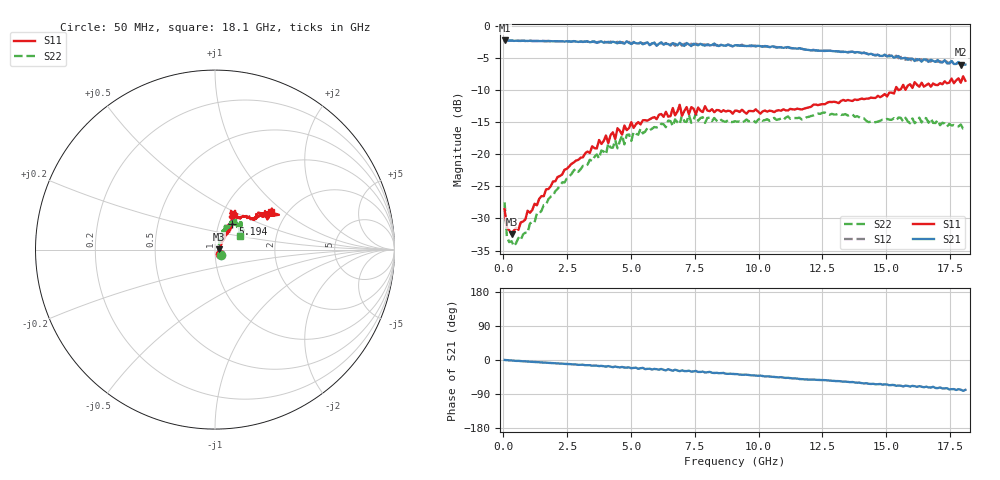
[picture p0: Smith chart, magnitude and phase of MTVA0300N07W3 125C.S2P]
! Network Analyzer HP8720D.06.14 Serial No. US36140669
!  7 Jul 2005  12:08:13
! Frequency  S11  S21  S12  S22
# HZ  S  DB R 50
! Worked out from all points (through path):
!   201 points, 50 MHz to 18.1 GHz, reference 50 ohm
!   highest |S21| = -2.25 dB at 50 MHz (marker M1); lowest = -6.0 dB at 17.92 GHz (marker M2)
!   group delay of S21, straight-line fit = 12.2 ps
!   lowest |S11| = -32.5 dB at 320.8 MHz (marker M3), VSWR 1.05, Z = 52.4 + j0.113 ohm
!   |S11| at or under -10 dB: start of sweep to 15.35 GHz
!   |S22| runs from -34.3 to -13.5 dB; largest |S21 - S12| = 0.042
!   S11 on the Smith chart (normalised r, x): 50 MHz: 1.06, -0.05; 5.194 GHz: 1.16, +0.34; 18.1 GHz: 1.67, +0.80
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5e7  -28.58 -40.6  -2.25 0.2  -2.27 0.3  -27.49 -40.4
1.4025e8  -31.43 -21.5  -2.33 -0.4  -2.31 -0.5  -32.89 -25.3
3.2075e8  -32.46 2.6  -2.25 -1.1  -2.28 -1.1  -33.55 -0.8
6.8175e8  -30.62 23.2  -2.32 -3.0  -2.30 -3.1  -33.39 28.2
2.30625e9  -23.14 48.3  -2.38 -9.6  -2.37 -9.8  -24.38 62.0
3.1185e9  -20.46 53.8  -2.46 -12.4  -2.48 -12.9  -21.80 65.2
4.11125e9  -18.27 57.4  -2.47 -16.1  -2.58 -17.5  -18.29 63.3
4.47225e9  -15.93 53.6  -2.69 -18.6  -2.46 -17.8  -19.07 68.1
4.65275e9  -16.93 54.0  -2.64 -18.3  -2.51 -20.0  -17.03 67.3
5.19425e9  -15.32 55.3  -2.68 -20.3  -2.50 -20.9  -16.79 66.7
6.09675e9  -13.83 59.0  -2.75 -25.6  -2.64 -25.3  -15.69 59.0
6.7285e9  -13.93 65.8  -2.78 -25.5  -3.07 -26.4  -14.55 54.2
6.909e9  -12.27 62.6  -2.61 -29.4  -2.69 -27.5  -15.31 54.8
6.99925e9  -13.96 62.6  -2.87 -27.4  -3.06 -29.7  -13.89 55.3
7.36025e9  -12.66 57.8  -3.13 -30.5  -2.76 -29.7  -15.10 58.7
7.54075e9  -13.77 60.7  -2.87 -28.8  -2.75 -32.0  -13.64 57.1
7.90175e9  -12.51 62.9  -3.05 -32.9  -2.89 -31.2  -15.11 53.0
9.075e9  -13.19 62.7  -3.00 -37.1  -2.97 -37.2  -14.85 47.2
1.21435e10  -12.27 50.0  -3.76 -51.7  -3.71 -51.9  -13.94 47.5
1.512175e10  -10.39 37.1  -4.71 -66.7  -4.51 -66.1  -14.61 40.9
1.79195e10  -8.84 31.3  -6.01 -78.4  -5.81 -79.3  -15.35 35.6
1.81e10  -8.52 33.5  -6.01 -78.8  -6.26 -79.7  -15.99 29.5
